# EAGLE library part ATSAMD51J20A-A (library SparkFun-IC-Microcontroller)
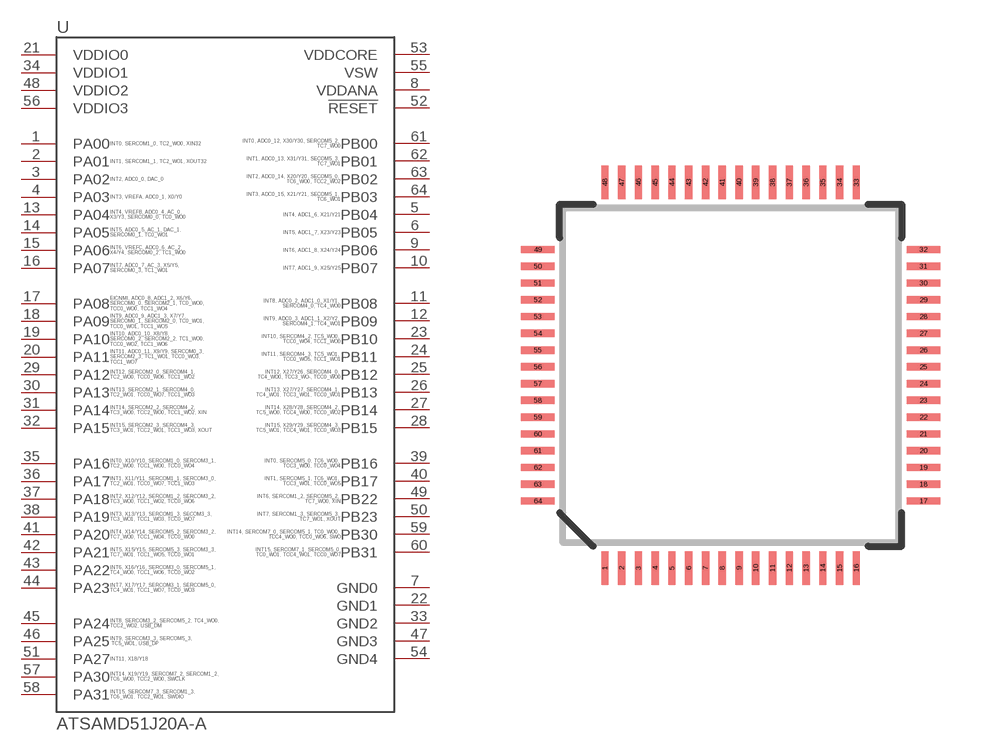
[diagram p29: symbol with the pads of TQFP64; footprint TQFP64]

Designator prefix U

## ATSAMD51J20A-A (PROD_ID: IC-13952)  [TQFP64]
1  PA00
2  PA01
3  PA02
4  PA03
5  PB04
6  PB05
7  GND0
8  VDDANA
9  PB06
10  PB07
11  PB08
12  PB09
13  PA04
14  PA05
15  PA06
16  PA07
17  PA08
18  PA09
19  PA10
20  PA11
21  VDDIO0
22  GND1
23  PB10
24  PB11
25  PB12
26  PB13
27  PB14
28  PB15
29  PA12
30  PA13
31  PA14
32  PA15
33  GND2
34  VDDIO1
35  PA16
36  PA17
37  PA18
38  PA19
39  PB16
40  PB17
41  PA20
42  PA21
43  PA22
44  PA23
45  PA24
46  PA25
47  GND3
48  VDDIO2
49  PB22
50  PB23
51  PA27
52  !RESET
53  VDDCORE
54  GND4
55  VSW
56  VDDIO3
57  PA30
58  PA31
59  PB30
60  PB31
61  PB00
62  PB01
63  PB02
64  PB03

## Footprint TQFP64 (pad centres in mm)
64-Lead TQFP Plastic Thin Quad Flatpack - 10x10x1mm Body, 2mmFP
smd 0.22 x 1: 1 -3.75,-5.75; 2 -3.25,-5.75; 3 -2.75,-5.75; 4 -2.25,-5.75; 5 -1.75,-5.75; 6 -1.25,-5.75; 7 -0.75,-5.75; 8 -0.25,-5.75; 9 0.25,-5.75; 10 0.75,-5.75; 11 1.25,-5.75; 12 1.75,-5.75; 13 2.25,-5.75; 14 2.75,-5.75; 15 3.25,-5.75; 16 3.75,-5.75; 33 3.75,5.75; 34 3.25,5.75; 35 2.75,5.75; 36 2.25,5.75; 37 1.75,5.75; 38 1.25,5.75; 39 0.75,5.75; 40 0.25,5.75; 41 -0.25,5.75; 42 -0.75,5.75; 43 -1.25,5.75; 44 -1.75,5.75; 45 -2.25,5.75; 46 -2.75,5.75; 47 -3.25,5.75; 48 -3.75,5.75
smd 1 x 0.22: 17 5.75,-3.75; 18 5.75,-3.25; 19 5.75,-2.75; 20 5.75,-2.25; 21 5.75,-1.75; 22 5.75,-1.25; 23 5.75,-0.75; 24 5.75,-0.25; 25 5.75,0.25; 26 5.75,0.75; 27 5.75,1.25; 28 5.75,1.75; 29 5.75,2.25; 30 5.75,2.75; 31 5.75,3.25; 32 5.75,3.75; 49 -5.75,3.75; 50 -5.75,3.25; 51 -5.75,2.75; 52 -5.75,2.25; 53 -5.75,1.75; 54 -5.75,1.25; 55 -5.75,0.75; 56 -5.75,0.25; 57 -5.75,-0.25; 58 -5.75,-0.75; 59 -5.75,-1.25; 60 -5.75,-1.75; 61 -5.75,-2.25; 62 -5.75,-2.75; 63 -5.75,-3.25; 64 -5.75,-3.75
